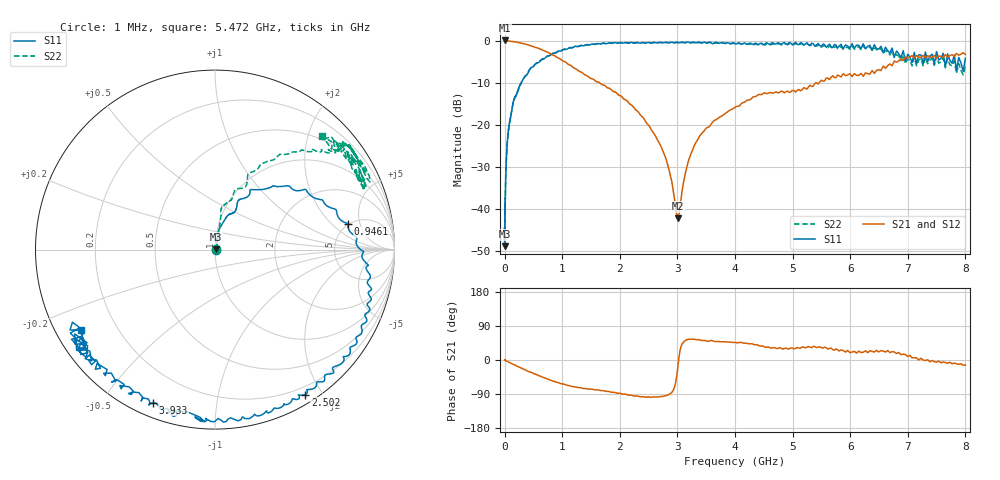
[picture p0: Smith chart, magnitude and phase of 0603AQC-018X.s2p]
!s-Parameter Generated by FASTRON Sdn. Bhd.
!FASTRON P/N : 0603AQC-018X
!Keysight Technologies: E5071C_MY46733604_B.14.02
!Date: Thu Jun 25 13:52:20 2026
!Version  :Rev00  Thu Jun 25 13:52:20 2026
!Data & Calibration Information:
!Freq  S11:SOLT2(ON)  S21:SOLT2(ON)  S12:SOLT2(ON)  S22:SOLT2(ON)
!PortZ  Port1:50+j0  Port2:50+j0
!When reading reference impedance value at option line is always used.
! Remarks : This data is being provided solely for informational purposes.
# Hz S dB R 50
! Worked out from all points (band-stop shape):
!   1601 points, 1 MHz to 8 GHz, reference 50 ohm
!   highest |S21| = 0.03 dB at 6.912 MHz (marker M1); lowest = -42.2 dB at 3.015 GHz (marker M2)
!   |S21| within 3 dB of the highest: start of sweep to 778.9 MHz; 7.950609 GHz to 7.970803 GHz (20.19 MHz wide, 0.254 % of centre)
!   lowest |S11| = -48.8 dB at 1.605 MHz (marker M3), VSWR 1.01, Z = 50.4 + j0.0977 ohm
!   |S11| at or under -10 dB: start of sweep to 290.9 MHz
!   |S22| runs from -47.7 to -0.4 dB; largest |S21 - S12| = 0.011
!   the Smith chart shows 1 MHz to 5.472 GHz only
!   S11 on the Smith chart (normalised r, x): 1 MHz: 1.01, +0.00; 946.1 MHz: 4.96, +3.26; 2.502 GHz: 0.11, -1.80; 3.933 GHz: 0.06, -0.67; 5.472 GHz: 0.07, -0.28
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1000000  -45.90 4.0  -0.05 -0.2  -0.05 -0.1  -45.50 12.9
1604653  -48.80 15.5  -0.05 -0.2  -0.05 -0.1  -46.90 0.3
4479405  -43.10 47.0  -0.05 -0.4  -0.05 -0.4  -43.20 53.1
6911657  -40.10 42.6  0.03 -1.1  -0.02 -0.5  -39.90 51.2
1.345746e7  -37.40 70.3  -0.05 -1.1  -0.06 -1.2  -35.90 69.4
2.00676e7  -32.50 69.2  -0.06 -1.7  -0.07 -1.6  -32.20 79.6
8.994653e7  -19.20 79.4  -0.13 -7.0  -0.14 -7.0  -19.40 78.3
4.006501e8  -7.87 55.6  -0.95 -29.1  -0.95 -29.1  -7.74 64.3
6.54293e8  -4.36 33.6  -2.21 -44.7  -2.20 -44.7  -4.50 57.1
9.461178e8  -2.44 10.8  -4.20 -60.4  -4.20 -60.6  -2.58 47.8
1.7949e9  -0.60 -28.6  -11.20 -82.8  -11.30 -83.0  -0.61 39.3
2.501569e9  -0.43 -58.1  -20.10 -97.5  -20.10 -97.6  -0.50 34.8
2.721653e9  -0.49 -65.9  -25.30 -96.6  -25.30 -96.7  -0.51 37.0
2.941737e9  -0.50 -72.2  -36.80 -75.2  -36.80 -75.1  -0.47 37.2
3.015098e9  -0.43 -76.2  -42.20 -8.3  -42.00 -8.4  -0.48 37.8
3.365624e9  -0.36 -90.2  -23.20 53.8  -23.20 53.8  -0.47 31.2
3.933151e9  -0.73 -112.0  -16.40 46.8  -16.40 46.7  -0.71 32.2
4.744521e9  -0.49 -140.0  -12.40 30.5  -12.40 30.2  -0.79 22.4
5.472309e9  -1.21 -149.0  -9.81 35.1  -9.80 34.8  -1.20 46.7
6.419251e9  -0.97 -175.0  -7.78 21.1  -7.76 20.6  -1.74 43.9
7.151793e9  -5.55 170.0  -3.49 5.7  -3.48 4.8  -5.99 43.6
8e9  -4.22 138.0  -3.30 -13.1  -3.33 -13.8  -5.99 45.3
